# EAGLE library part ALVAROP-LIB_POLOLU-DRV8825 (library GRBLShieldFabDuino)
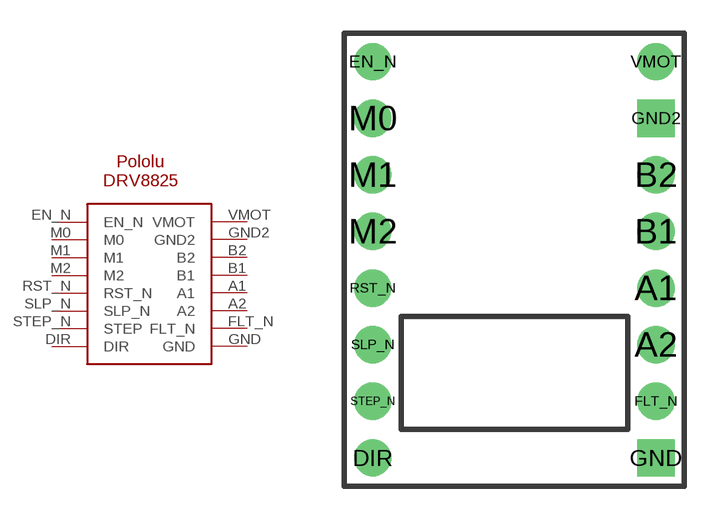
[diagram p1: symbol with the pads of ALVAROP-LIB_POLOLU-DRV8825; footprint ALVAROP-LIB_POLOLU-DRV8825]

Designator prefix -

## ALVAROP-LIB_POLOLU-DRV8825  [ALVAROP-LIB_POLOLU-DRV8825]
A1  A1
A2  A2
B1  B1
B2  B2
DIR  DIR
EN_N  EN_N
FLT_N  FLT_N
GND  GND
GND2  GND2
M0  M0
M1  M1
M2  M2
RST_N  RST_N
SLP_N  SLP_N
STEP_N  STEP
VMOT  VMOT

## Footprint ALVAROP-LIB_POLOLU-DRV8825 (pad centres in mm)
drill 0.8 pad 1.676: A1 6.35,-1.27; A2 6.35,-3.81; B1 6.35,1.27; B2 6.35,3.81; DIR -6.35,-8.89; EN_N -6.35,8.89; FLT_N 6.35,-6.35; M0 -6.35,6.35; M1 -6.35,3.81; M2 -6.35,1.27; RST_N -6.35,-1.27; SLP_N -6.35,-3.81; STEP_N -6.35,-6.35; VMOT 6.35,8.89
drill 0.8 pad 1.676 square: GND 6.35,-8.89; GND2 6.35,6.35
